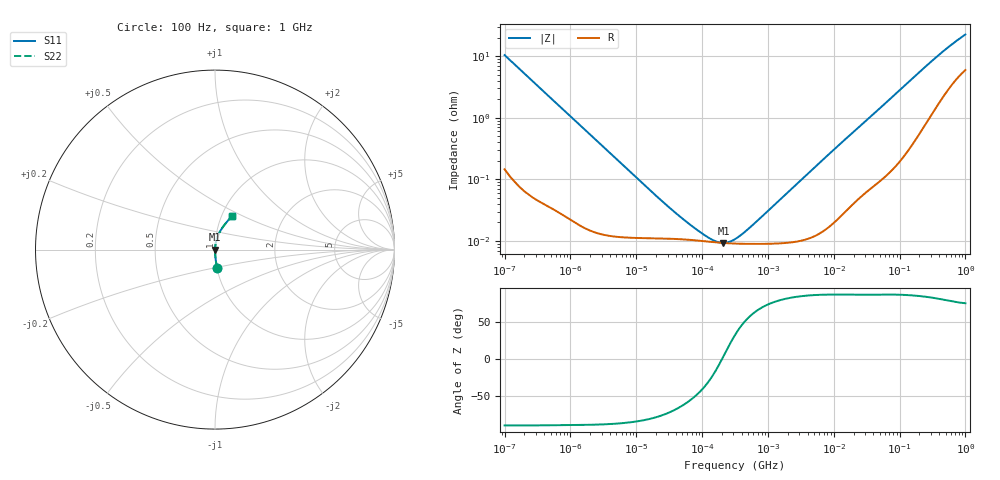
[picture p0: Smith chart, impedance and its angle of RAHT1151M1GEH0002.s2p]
! RAHT1151M1GEH0002  S-PARAMETER MODEL  (AEC-Q200 qualified)
! Model Generated by ELNA Corporation (http://www.ty-top.com)
! Version 1.0
! ELNA Control No. 201214
! Copyright (c) 2020 ELNA CO.,LTD. All Rights Reserved.
! Products Name : CONDUCTIVE POLYMER HYBRID ALUMINUM ELECTROLYTIC CAPACITORS
! Characteristics :
!  Capacitance  :  150uF  ,  Rated voltage  :  35V
!  Operating Temp. Range  :  -55 to +105 degC  ,  Endurance  :  5000hr at 105 degC
!  Dimension D  :  8mm  ,  Dimension L  :  10mm
! Frequency Range : 100Hz - 1GHz
! External Node Assignments :
!  1  o---| |---o  2
# MHz S RI R 50
!Freq[MHz].  S11 Real  S11 Imag  S21 Real  S21 Imag  S12 Real  S12 Imag  S22 Real  S22 Imag
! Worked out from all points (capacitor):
!   401 points, 100 Hz to 1 GHz, reference 50 ohm
!   read as one part in series: C = 152 uF near 108 Hz
!   lowest |Z| = 9.3 mohm at 211.3 kHz (marker M1)
!   series resonance near 201.7 kHz, so ESL is about 4.1 nH
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0.0001  0.0122 -0.1031  0.9878 0.1031  0.9878 0.1031  0.0122 -0.1031
0.000113  0.00971 -0.0917  0.9903 0.0917  0.9903 0.0917  0.00971 -0.0917
0.000183  0.00395 -0.0569  0.9961 0.0569  0.9961 0.0569  0.00395 -0.0569
0.000309  0.00161 -0.0339  0.9984 0.0339  0.9984 0.0339  0.00161 -0.0339
0.001488  0.000222 -0.00714  0.9998 0.00714  0.9998 0.00714  0.000222 -0.00714
0.022131  0.00011 -0.000479  0.9999 0.000479  0.9999 0.000479  0.00011 -0.000479
0.051582  0.000106 -0.0002  0.9999 0.0002  0.9999 0.0002  0.000106 -0.0002
0.110917  9.88e-05 -7.31e-05  0.9999 7.31e-05  0.9999 7.31e-05  9.88e-05 -7.31e-05
0.153109  9.55e-05 -3.29e-05  0.9999 3.29e-05  0.9999 3.29e-05  9.55e-05 -3.29e-05
0.211349  9.28e-05 5.64e-06  0.9999 -5.64e-06  0.9999 -5.64e-06  9.28e-05 5.64e-06
0.269153  9.14e-05 3.55e-05  0.9999 -3.55e-05  0.9999 -3.55e-05  9.14e-05 3.55e-05
0.316228  9.07e-05 5.67e-05  0.9999 -5.67e-05  0.9999 -5.67e-05  9.07e-05 5.67e-05
0.402717  9.01e-05 9.17e-05  0.9999 -9.17e-05  0.9999 -9.17e-05  9.01e-05 9.17e-05
0.578762  8.96e-05 0.000155  0.9999 -0.000155  0.9999 -0.000155  8.96e-05 0.000155
4.704354  0.000117 0.00143  0.9999 -0.00143  0.9999 -0.00143  0.000117 0.00143
12.8825  0.000269 0.00387  0.9997 -0.00387  0.9997 -0.00387  0.000269 0.00387
69.9842  0.00166 0.0197  0.9983 -0.0197  0.9983 -0.0197  0.00166 0.0197
176.8072  0.00679 0.0483  0.9932 -0.0483  0.9932 -0.0483  0.00679 0.0483
380.1894  0.0254 0.0961  0.9746 -0.0961  0.9746 -0.0961  0.0254 0.0961
668.3439  0.059 0.1459  0.941 -0.1459  0.941 -0.1459  0.059 0.1459
922.5714  0.0869 0.1777  0.9131 -0.1777  0.9131 -0.1777  0.0869 0.1777
1000  0.0946 0.1861  0.9054 -0.1861  0.9054 -0.1861  0.0946 0.1861
